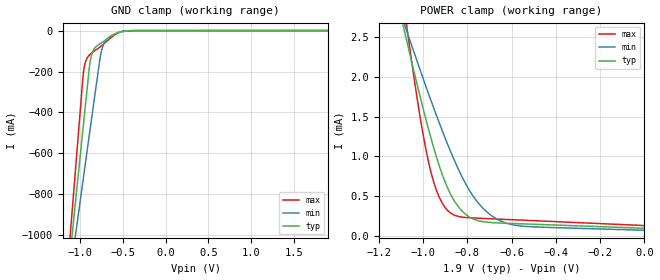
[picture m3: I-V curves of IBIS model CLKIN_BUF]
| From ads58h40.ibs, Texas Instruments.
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|   Model CLKIN_BUF
[Model]  CLKIN_BUF
Model_type Terminator
C_comp   2.5000pF   2.2500pF   2.7500pF
[Temperature Range]   25.0000   0.1250k   -40.0000
[Voltage Range]   1.9000V   1.8000V   2.0000V
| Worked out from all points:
|   GND clamp passes 1 mA (typ) near -0.45 V on its own axis
|   POWER clamp passes 1 mA (typ) near -0.94 V on its own axis
[GND_clamp]
|Voltage   I(typ)   I(min)   I(max)
-1.9V     -4.338A    -3.616A    -5.134A
-1.17V    -1.322A    -1.362A    -1.298A
-1.07V    -913mA     -1.056A    -775.9mA
-970mV    -504.8mA   -751.8mA   -255mA
-940mV    -382.7mA   -660.7mA   -159.7mA
-890mV    -180.4mA   -509.2mA   -119.8mA
-860mV    -113.1mA   -418.7mA   -108.8mA
-750mV    -60.17mA   -102.6mA   -75.09mA
-710mV    -48.74mA   -56.35mA   -60.84mA
-640mV    -28.61mA   -26.55mA   -35.41mA
-430mV    -687.1uA   -1.149mA   -618.1uA
1.9V      95.72uA    78.57uA    117.4uA
[POWER_clamp]
|Voltage   I(typ)   I(min)   I(max)
-1.9V     13.36mA    9.872mA    22.13mA
-1.09V    2.656mA    2.717mA    2.983mA
-1.08V    2.535mA    2.634mA    2.775mA
-1.07V    2.415mA    2.552mA    2.571mA
-1.01V    1.72mA     2.065mA    1.446mA
-970mV    1.291mA    1.751mA    869.3uA
-930mV    912.1uA    1.448mA    508.9uA
-880mV    550.4uA    1.094mA    297.2uA
-820mV    303.9uA    723.5uA    235.3uA
-760mV    198.2uA    447.8uA    223.6uA
-640mV    160.3uA    176.4uA    208.5uA
0V        95.72uA    70.35uA    129.7uA
